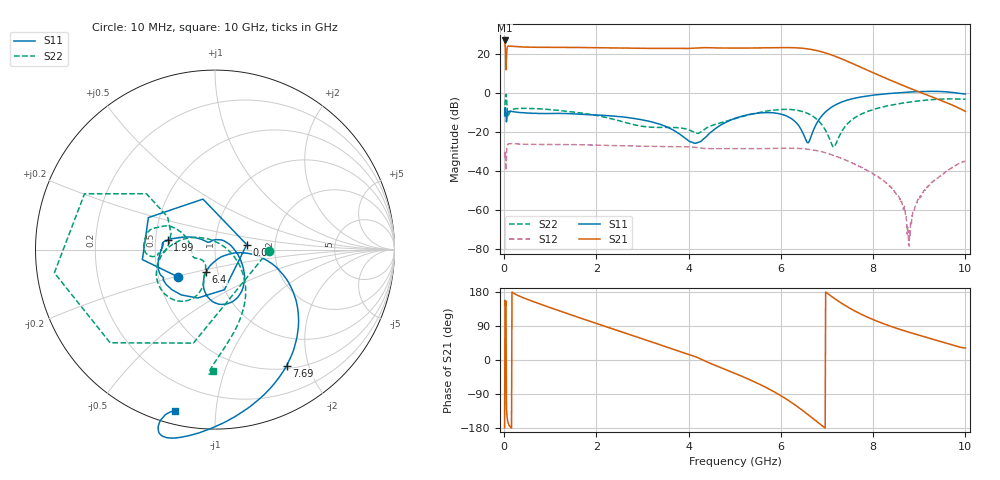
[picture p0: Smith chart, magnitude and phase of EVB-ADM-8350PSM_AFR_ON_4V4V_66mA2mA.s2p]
!Keysight Technologies,N5247B,US58420632,A.15.75.19
!Date: Monday, January 30, 2023 13:27:27
!Correction: S11(C  2-Port  )
!S21(C  2-Port  )
!S12(C  2-Port  )
!S22(C  2-Port  )
!S2P File: Measurements: S11, S21, S12, S22:
# Hz S  dB  R 50
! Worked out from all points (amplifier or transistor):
!   1000 points, 10 MHz to 10 GHz, reference 50 ohm
!   highest |S21| = 26.7 dB at 10 MHz (marker M1)
!   |S21| within 3 dB of that: 78.66 MHz to 168.9 MHz (90.26 MHz wide, 72.9 % of centre)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
!   unconditionally stable (mu >= 1): 33.28 MHz to 825.9 MHz; 2.384 GHz to 5.629 GHz; 6.131 GHz to 8.545 GHz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
!   at 1.67 GHz: K = 0.97, MSG = 24.9 dB, |S12| = -26.6 dB
!   at 5.01 GHz: K = 1.11, MAG = 23.7 dB, |S12| = -28.7 dB
!   at 10 GHz: K = 5.94, MAG = 2.0 dB, |S12| = -35.0 dB
!   S11 on the Smith chart (normalised r, x): 10 MHz: 0.63, -0.21; 50 MHz: 1.43, +0.08; 1.99 GHz: 0.58, +0.07; 6.4 GHz: 0.88, -0.23; 7.69 GHz: 0.54, -1.66; 10 GHz: 0.06, -0.78
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1e7  -11.84 -143.5  26.71 -179.1  -33.25 76.0  -10.49 -1.4
5e7  -14.95 8.9  17.79 -128.7  -33.08 82.1  -2.04 156.9
8e7  -10.04 -126.7  23.76 -162.8  -26.47 38.5  -11.66 159.9
1e8  -9.52 -144.3  23.87 -170.5  -26.17 27.2  -11.26 179.9
1.3e8  -9.51 -155.0  23.77 -175.9  -26.11 18.2  -9.85 -174.4
2.3e8  -9.87 -168.9  23.59 174.5  -26.17 4.3  -8.29 -177.1
6.1e8  -10.55 179.0  23.24 155.2  -26.41 -15.1  -8.11 169.1
1.68e9  -11.08 170.0  23.10 109.5  -26.67 -51.4  -10.45 153.8
1.99e9  -11.41 168.6  22.99 96.8  -26.83 -61.2  -11.56 152.2
2.65e9  -12.61 164.3  22.77 70.0  -27.19 -82.8  -15.38 158.2
3.34e9  -15.91 154.0  22.64 41.8  -27.52 -105.7  -17.77 -171.7
4.31e9  -23.93 58.9  23.03 -0.0  -28.45 -143.6  -19.34 -118.8
5.01e9  -13.10 -42.0  22.79 -35.6  -28.65 -167.5  -13.25 -108.8
5.86e9  -10.37 -86.8  23.03 -84.3  -28.45 154.8  -8.87 -128.7
6.14e9  -12.11 -102.3  23.07 -104.8  -28.41 138.8  -8.56 -143.3
6.4e9  -17.35 -111.4  22.85 -126.8  -28.55 121.4  -9.23 -160.6
6.67e9  -21.36 -16.5  22.07 -152.1  -29.18 101.3  -11.75 177.2
7.16e9  -6.54 -26.1  18.77 162.5  -32.27 65.1  -27.56 48.5
7.69e9  -2.38 -58.3  13.47 123.8  -37.74 35.9  -11.55 -50.1
8.34e9  -0.44 -85.1  6.71 90.7  -47.19 13.7  -6.61 -76.5
8.78e9  0.31 -96.6  2.42 73.2  -78.52 -24.6  -4.82 -86.5
1e10  -0.67 -104.1  -9.52 31.4  -35.03 117.3  -3.37 -90.9
